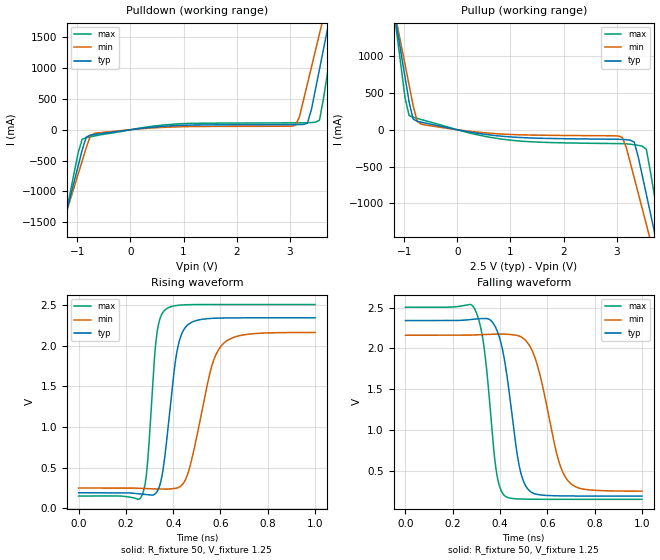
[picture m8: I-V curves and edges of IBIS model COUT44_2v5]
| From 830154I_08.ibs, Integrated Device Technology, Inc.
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[Model] COUT44_2v5
Model_type   Output
Polarity   Non-Inverting
Vmeas = 1.25
Rref = 50
Cref = 0
Vref = 1.25
|   typ   min   max
C_comp   2pF   1.5pF   2.5pF
|   typ   min   max
[Voltage range]  2.5V   2.375V   2.625V
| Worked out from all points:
|   slope of the pulldown table from 0 to 0.375 V, typ, clamps not added: 9.8 ohm
|   slope of the pullup table from 0 to 0.375 V, typ, clamps not added: 7.87 ohm
|   rising waveform, R_fixture 50, V_fixture 1.25: 20-80 % time 51.1ps typ, 85.4ps min, 33.2ps max; typ from 0.189 V to 2.34 V
|   falling waveform, R_fixture 50, V_fixture 1.25: 20-80 % time 61.7ps typ, 87.5ps min, 47ps max; typ from 2.34 V to 0.189 V
[pulldown]
|Voltage   I (typ)   I (min)   I (max)
-2.5V     -5.69A     -4.969A    -6.868A
-1.288V   -1.607A    -1.566A    -1.677A
-909.1mV  -327.6mA   -504mA     -152.8mA
-833.3mV  -120.4mA   -292.2mA   -129.9mA
-681.8mV  -77.5mA    -59.86mA   -102.3mA
833.3mV   66.73mA    45.82mA    91.42mA
3.106V    83.18mA    71.08mA    112mA
3.333V    106.9mA    744.6mA    113.9mA
3.561V    980.4mA    1.557A     155.3mA
3.712V    1.634A     2.1A       924.4mA
3.864V    2.289A     2.645A     1.762A
5V        7.244A     6.759A     8.095A
[pullup]
|Voltage   I (typ)   I (min)   I (max)
-2.5V     7.371A     6.419A     8.931A
-1.136V   1.375A     1.435A     1.282A
-909.1mV  376.1mA    606.7mA    193mA
-833.3mV  145.3mA    330.7mA    169.8mA
-681.8mV  102.9mA    76.06mA    138.9mA
3.106V    -131.6mA   -102.3mA   -188.9mA
3.333V    -169mA     -656.2mA   -203.7mA
3.561V    -877.5mA   -1.285A    -266.1mA
3.636V    -1.131A    -1.496A    -564.3mA
3.712V    -1.384A    -1.706A    -887.8mA
3.864V    -1.891A    -2.128A    -1.535A
5V        -5.702A    -5.301A    -6.39A
[Ramp]
|   typ   min   max
dV/dt_r   1.742/.0817n   1.542/.134n   1.911/.0544p
dV/dt_f   1.742/.0987n   1.542/.138n   1.911/.0762p
[Rising Waveform]
R_fixture = 50
V_fixture = 1.25
V_fixture_max = 1.3125
V_fixture_min = 1.1875
C_fixture = 0.0p
| Time   typ   min   max
0s        189.4mV    248.4mV    149.4mV
267.3ps   174.3mV    243.5mV    152.5mV
290.4ps   167mV      240.4mV    520.7mV
330ps     196.3mV    236.4mV    2.122V
367.4ps   703.5mV    234.6mV    2.444V
414.7ps   1.907V     247.2mV    2.493V
460.9ps   2.253V     416.6mV    2.503V
558.8ps   2.334V     1.702V     2.505V
606.1ps   2.339V     2.006V     2.505V
999.9ps   2.342V     2.161V     2.505V
[Falling Waveform]
R_fixture = 50
V_fixture = 1.25
V_fixture_max = 1.3125
V_fixture_min = 1.1875
C_fixture = 0.0p
| Time   typ   min   max
0s        2.342V     2.162V     2.505V
292.6ps   2.36V      2.165V     2.484V
332.2ps   2.367V     2.17V      2.016V
385ps     2.233V     2.177V     478.8mV
420.2ps   1.832V     2.175V     191.3mV
478.5ps   597.7mV    2.154V     153.9mV
523.6ps   256.6mV    2.038V     150.7mV
645.7ps   192.2mV    642.9mV    149.5mV
684.2ps   190.8mV    388.5mV    149.4mV
999.9ps   189.4mV    249.4mV    149.4mV
